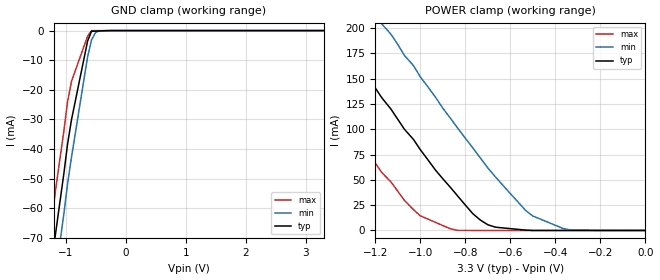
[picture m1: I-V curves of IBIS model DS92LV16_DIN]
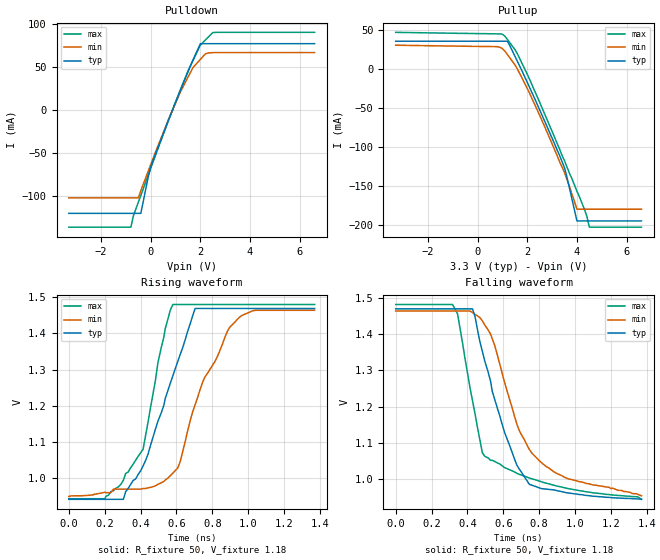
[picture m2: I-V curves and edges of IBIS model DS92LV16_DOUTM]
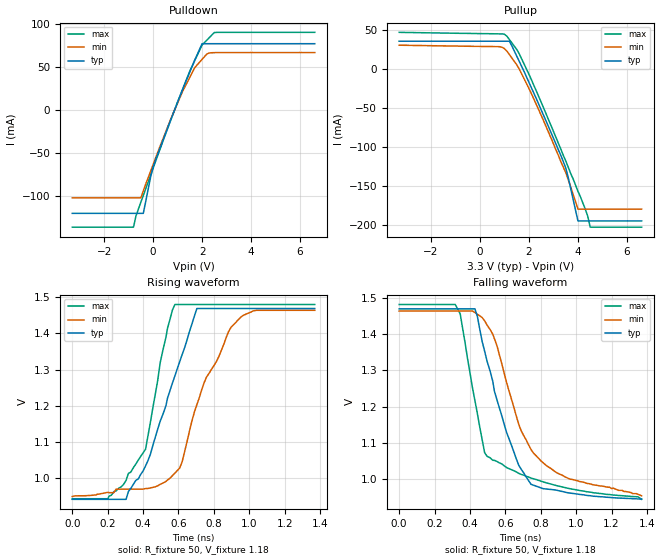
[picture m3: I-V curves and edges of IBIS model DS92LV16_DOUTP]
|   National Semiconductor Corporation
|   IBIS Model of DS92LV16TVHG
|   16-Bit BUS LVDS Serializer/Deserializer
|   80 Lead PQFP Package
[IBIS Ver]   3.2
[Comment Char]   |_char
[File name]   ds92lv16tvhg.ibs
[File Rev]   1.5
[Date]   03/22/04
[Source]
SPICE to IBIS Translation
[Notes]
Created by Tim Coyle; dglisic for Revs 1.4 and beyond.
Rev 1.5: - Updated RINP and RINM models.
Rev 1.4: - Changed Cref to 15pF, to match the datasheet value.
Rev 1.3: - Fixed V-T time scale for LVDS output data
   - Modified pull-up data for LVDS output data to make more accurate
   - Accounted for power/ground clamp data in output models
Rev 1.2: - Changed Ramp values in accordance with IBIS specification
Rev 1.1: - Changed RCLK and LOCK pins to output model types
   - Added typ min max description to Ramp data for clarification
[Disclaimer]
(C) Copyright National Semiconductor Corporation 2002
   All rights reserved
   National Semiconductor Corporation hereby grants
the user of this IBIS model a non-exclusive, nontransferable
license to use this IBIS model under the following terms.
Before using this IBIS model, the user should read this
license.  If the user does not accept these terms,  the
IBIS model should be returned to National within 30 days.
   The user is granted this license only to use the
IBIS model and is not granted rights to sell, load, rent,
lease or license the IBIS model in whole or in part, or in
modified form to anyone other than user. User may modify
the IBIS model to suit its specific applications but rights
to derivative works and such modifications shall belong to
National.
   This IBIS model is provided on an "AS IS" basis and
National makes absolutely no warranty with respect to the
information contained herein.NATIONAL DISCLAIMS AND CUSTOMER
WAIVES ALL WARRANTIES, EXPRESS OR IMPLIED, INCLUDING
WARRANTIES OF MERCHANTABILITY OR FITNESS FOR A PARTICULAR
PURPOSE. The entire risk as to quality and performance is
with the Customer. ACCORDINGLY, IN NO EVENT SHALL THE
COMPANY BE LIABLE FOR ANY DAMAGES, WHETHER IN CONTRACT OR
TORT,INCLUDING ANY LOST PROFITS OR OTHER INCIDENTAL,
CONSEQUENTIAL, EXEMPLARY, OR PUNITIVE DAMAGES ARISING OUT
OF THE USE OR APPLICATION OF THE IBIS model provided in
this package.Further, National reserves the right to make
changes without notice to any product herein to improve
reliability, function, or design. National does not convey
any license under patent rights or any other intellectual
property rights, including those of third parties.
   National is not obligated to provide maintenance or support
for the licensed IBIS model.
Contact National at ATTN:INTERFACE APPLICATIONS/IBIS MODELS.
5 Foden Road, M/S 03-03, South Porltand, ME 04106
(207) 541-8203
[Copyright]
(c) Copyright 2002 National Semiconductor Corp.
[Component]   DS92LV16
Si_location Pin
Timing_location Pin
[Manufacturer]   National Semiconductor Corp.
[Package]
|   TYP   MIN   MAX
R_pkg   50.0m   50.0m   50.0m
L_pkg   1.164nH   1.04n   1.33n
C_pkg   0.207pF   0.178p   0.245p
[Pin]   signal_name   model_name   R_pin   L_pin   C_pin
1   RPWDN   DS92LV16_CONTROL   50.0m   1.33n   0.245p
2   REN   DS92LV16_CONTROL   50.0m   1.04n   0.178p
3   CONFIG1 DS92LV16_CONTROL   50.0m   1.04n   0.178p
4   REFCLK  DS92LV16_CONTROL   50.0m   1.04n   0.178p
5   AVDD   POWER   50.0m   1.33n   0.245p
6   AGND   GND   50.0m   1.04n   0.178p
7   RINP   DS92LV16_RINP   50.0m   1.04n   0.178p
8   RINM   DS92LV16_RINM   50.0m   1.33n   0.245p
9   AGND   GND   50.0m   1.33n   0.245p
10   AVDD   POWER   50.0m   1.33n   0.245p
11   AVDD   POWER   50.0m   1.33n   0.245p
12   AGND   GND   50.0m   1.33n   0.245p
13   DOUTP   DS92LV16_DOUTP   50.0m   1.33n   0.245p
14   DOUTM   DS92LV16_DOUTM   50.0m   1.33n   0.245p
15   AVDD   POWER   50.0m   1.33n   0.245p
16   AGND   GND   50.0m   1.33n   0.245p
17   TCLK   DS92LV16_CONTROL   50.0m   1.33n   0.245p
18   CONFIG2 DS92LV16_CONTROL   50.0m   1.33n   0.245p
19   DEN   DS92LV16_CONTROL   50.0m   1.33n   0.245p
20   SYNC   DS92LV16_CONTROL   50.0m   1.33n   0.245p
21   DIN0   DS92LV16_DIN   50.0m   1.33n   0.245p
22   DIN1   DS92LV16_DIN   50.0m   1.33n   0.245p
23   DIN2   DS92LV16_DIN   50.0m   1.33n   0.245p
24   DIN3   DS92LV16_DIN   50.0m   1.33n   0.245p
25   DIN4   DS92LV16_DIN   50.0m   1.33n   0.245p
26   DIN5   DS92LV16_DIN   50.0m   1.33n   0.245p
27   DIN6   DS92LV16_DIN   50.0m   1.33n   0.245p
28   DIN7   DS92LV16_DIN   50.0m   1.33n   0.245p
29   PGND   GND   50.0m   1.33n   0.245p
30   PVDD   POWER   50.0m   1.33n   0.245p
31   PVDD   POWER   50.0m   1.33n   0.245p
32   PGND   GND   50.0m   1.33n   0.245p
33   DIN8   DS92LV16_DIN   50.0m   1.33n   0.245p
34   DIN9   DS92LV16_DIN   50.0m   1.33n   0.245p
35   DIN10   DS92LV16_DIN   50.0m   1.33n   0.245p
36   DIN11   DS92LV16_DIN   50.0m   1.33n   0.245p
37   DIN12   DS92LV16_DIN   50.0m   1.33n   0.245p
38   DIN13   DS92LV16_DIN   50.0m   1.33n   0.245p
39   DIN14   DS92LV16_DIN   50.0m   1.33n   0.245p
40   DIN15   DS92LV16_DIN   50.0m   1.33n   0.245p
41   DGND   GND   50.0m   1.33n   0.245p
42   TPWDN   DS92LV16_CONTROL   50.0m   1.33n   0.245p
43   DVDD   POWER   50.0m   1.33n   0.245p
44   DGND   GND   50.0m   1.33n   0.245p
45   ROUT0   DS92LV16_ROUT   50.0m   1.33n   0.245p
46   ROUT1   DS92LV16_ROUT   50.0m   1.33n   0.245p
47   ROUT2   DS92LV16_ROUT   50.0m   1.33n   0.245p
48   ROUT3   DS92LV16_ROUT   50.0m   1.33n   0.245p
49   RCLK   DS92LV16_ROUT   50.0m   1.33n   0.245p
50   DVDD   POWER   50.0m   1.33n   0.245p
51   DGND   GND   50.0m   1.33n   0.245p
52   DGND   GND   50.0m   1.33n   0.245p
53   DVDD   POWER   50.0m   1.33n   0.245p
54   ROUT4   DS92LV16_ROUT   50.0m   1.33n   0.245p
55   ROUT5   DS92LV16_ROUT   50.0m   1.33n   0.245p
56   ROUT6   DS92LV16_ROUT   50.0m   1.33n   0.245p
57   ROUT7   DS92LV16_ROUT   50.0m   1.33n   0.245p
58   DVDD   POWER   50.0m   1.33n   0.245p
59   DGND   GND   50.0m   1.33n   0.245p
60   DGND   GND   50.0m   1.33n   0.245p
61   DGND   GND   50.0m   1.33n   0.245p
62   DVDD   POWER   50.0m   1.33n   0.245p
63   LOCK   DS92LV16_ROUT   50.0m   1.33n   0.245p
64   ROUT8   DS92LV16_ROUT   50.0m   1.33n   0.245p
65   ROUT9   DS92LV16_ROUT   50.0m   1.33n   0.245p
66   ROUT10  DS92LV16_ROUT   50.0m   1.33n   0.245p
67   ROUT11  DS92LV16_ROUT   50.0m   1.33n   0.245p
68   DGND   GND   50.0m   1.33n   0.245p
69   DVDD   POWER   50.0m   1.33n   0.245p
70   ROUT12  DS92LV16_ROUT   50.0m   1.33n   0.245p
71   ROUT13  DS92LV16_ROUT   50.0m   1.33n   0.245p
72   ROUT14  DS92LV16_ROUT   50.0m   1.33n   0.245p
73   ROUT15  DS92LV16_ROUT   50.0m   1.33n   0.245p
74   PGND   GND   50.0m   1.33n   0.245p
75   PVDD   POWER   50.0m   1.33n   0.245p
76   PGND   GND   50.0m   1.33n   0.245p
77   PVDD   POWER   50.0m   1.33n   0.245p
78   LINELE  DS92LV16_CONTROL   50.0m   1.33n   0.245p
79   LOCALLE DS92LV16_CONTROL   50.0m   1.33n   0.245p
80   DGND   GND   50.0m   1.33n   0.245p
[Diff Pin] inv_pin   vdiff   tdelay_typ   tdelay_min   tdelay_max
| The '+' pin is Diff_pin and the '-' pin is the inv_pin
| Receiver Vth = +/-100mV
7   8   0.1   0   0   0
13   14   NA   0   0   0
| Models and submodels in the file (7): DS92LV16_DIN (Input), DS92LV16_DOUTM (Output), DS92LV16_DOUTP (Output), DS92LV16_RINM (Input), DS92LV16_RINP (Input), DS92LV16_ROUT (Output), DS92LV16_CONTROL (Input)
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[Model]   DS92LV16_DIN
Model_type Input
Vinh=2.0
Vinl=0.8
C_comp   2.922pF   2.922pF   2.922pF
[Temperature Range] 25   85   -40
[Voltage Range]   3.3   3.15   3.45
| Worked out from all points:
|   GND clamp passes 1 mA (typ) near -0.58 V on its own axis
|   POWER clamp passes 1 mA (typ) near -0.56 V on its own axis
[GND Clamp]
|V(groundclamp)   I(typ)   I(min)   I(max)
-3.3V     -416mA     -429mA     -402mA
-1.3V     -89.7mA    -104mA     -74.9mA
-1.23V    -79.3mA    -93mA      -64.5mA
-1.17V    -69.1mA    -82.7mA    -54.4mA
-1.1V     -58.8mA    -72.5mA    -44.3mA
-1.03V    -48.6mA    -62.2mA    -34.2mA
-967mV    -38.4mA    -51.9mA    -24.1mA
-900mV    -30mA      -42.6mA    -17.1mA
-633mV    -3.57mA    -8.92mA    -1.9mA
-567mV    -239uA     -3.14mA    -420nA
-433mV    -133uA     -61.9uA    -233nA
3.3V      21.4pA     6.6nA      19.4pA
[POWER Clamp]
|Vtable   I(typ)   I(min)   I(max)
-3.3V     826mA      900mA      750mA
-1.63V    280mA      354mA      203mA
-1.6V     269mA      344mA      193mA
-1.37V    194mA      268mA      118mA
-1.17V    131mA      204mA      57.1mA
-1.13V    120mA      194mA      48mA
-1V       80mA       152mA      14.5mA
-833mV    33.9mA     101mA      60uA
-700mV    5.68mA     61.9mA     6.68uA
-533mV    372uA      20mA       1.71nA
-366mV    1.1uA      2.03mA     12.8pA
0V        6.66pA     6.59nA     6.3pA
[Model]   DS92LV16_DOUTM
Model_type Output
Polarity Inverting
Vref=1.20
Vmeas=1.20
Rref=50   | 100 Ohms Across Outputs OUTP and OUTM
Cref=5p
C_comp   3.122pF   3.122pF   3.122pF
[Temperature Range] 25   85   -40
[Voltage Range]   3.3   3.15   3.45
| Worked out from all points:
|   slope of the pulldown table from 0 to 0.495 V, typ, clamps not added: 13.1 ohm
|   falling waveform, R_fixture 50, V_fixture 1.18: 20-80 % time 190ps typ, 235ps min, 166ps max; typ from 1.47 V to 0.945 V
|   rising waveform, R_fixture 50, V_fixture 1.18: 20-80 % time 210ps typ, 224ps min, 147ps max; typ from 0.942 V to 1.47 V
[Pullup]
|Vtable   I(typ)   I(min)   I(max)
-3.3V     35mA       29.9mA     46.4mA
800mV     35mA       28mA       44.4mA
1.1V      35mA       22.3mA     41.4mA
1.2V      35mA       18mA       37.2mA
1.6V      9.43mA     -402uA     19.1mA
2.4V      -45.7mA    -52.9mA    -36mA
3.3V      -111mA     -119mA     -103mA
3.5V      -127mA     -133mA     -118mA
4V        -195mA     -180mA     -157mA
4.4V      -195mA     -180mA     -189mA
4.5V      -195mA     -180mA     -203mA
6.6V      -195mA     -180mA     -203mA
[Pulldown]
|V(pulldown)   I(typ)   I(min)   I(max)
-3.3V     -120mA     -102mA     -136mA
-800mV    -120mA     -102mA     -136mA
-700mV    -120mA     -102mA     -123mA
-500mV    -120mA     -102mA     -107mA
-400mV    -120mA     -93.8mA    -99.3mA
0V        -66.3mA    -63.4mA    -67.5mA
1.2V      23.4mA     21.4mA     23.8mA
1.7V      58mA       49.2mA     57.4mA
2V        77mA       58.8mA     75.5mA
2.2V      77mA       65.2mA     81.3mA
2.5V      77mA       66.6mA     90mA
6.6V      77mA       66.7mA     90.2mA
[Ramp]
|   typ   min   max
dV/dt_r   320mV/.213ns   310mV/.222ns   330mV/.150ns
dV/dt_f   320mv/.192ns   310mv/.241ns   330mv/.156ns
R_load=50
[Falling Waveform]
R_fixture=50
V_fixture=1.18
V_fixture_min=1.18
V_fixture_max=1.18
0s        1.47V      1.464V     1.482V
317ps     1.47V      1.464V     1.482V
345ps     1.47V      1.464V     1.456V
428ps     1.47V      1.46V      1.217V
497ps     1.325V     1.425V     1.063V
607ps     1.129V     1.267V     1.032V
676ps     1.038V     1.151V     1.016V
745ps     985.7mV    1.082V     1.003V
966ps     961.6mV    1V         973.5mV
1.37ns    945mV      954mV      944.3mV
[Rising Waveform]
R_fixture=50
V_fixture=1.18
V_fixture_min=1.18
V_fixture_max=1.18
0s        941.6mV    949.5mV    943.3mV
202ps     941.6mV    961.1mV    943.3mV
304ps     941.6mV    969.8mV    994mV
414ps     1.034V     971.4mV    1.08V
497ps     1.158V     983.1mV    1.32V
580ps     1.283V     1.014V     1.48V
704ps     1.469V     1.203V     1.48V
897ps     1.469V     1.417V     1.48V
1.04ns    1.469V     1.464V     1.48V
1.37ns    1.469V     1.464V     1.48V
[Model]   DS92LV16_DOUTP
Model_type Output
Polarity Non-Inverting
Vref=1.20
Vmeas=1.20
Rref=50   | 100 Ohms Across Outputs OUTP and OUTM
Cref=5p
C_comp   3.122pF   3.122pF   3.122pF
[Temperature Range] 25   85   -40
[Voltage Range]   3.3   3.15   3.45
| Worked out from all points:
|   slope of the pulldown table from 0 to 0.495 V, typ, clamps not added: 13.1 ohm
|   falling waveform, R_fixture 50, V_fixture 1.18: 20-80 % time 190ps typ, 235ps min, 166ps max; typ from 1.47 V to 0.945 V
|   rising waveform, R_fixture 50, V_fixture 1.18: 20-80 % time 210ps typ, 224ps min, 147ps max; typ from 0.942 V to 1.47 V
[Pullup]
|Vtable   I(typ)   I(min)   I(max)
-3.3V     35mA       29.9mA     46.4mA
800mV     35mA       28mA       44.4mA
1.1V      35mA       22.3mA     41.4mA
1.2V      35mA       18mA       37.2mA
1.6V      9.43mA     -402uA     19.1mA
2.4V      -45.7mA    -52.9mA    -36mA
3.3V      -111mA     -119mA     -103mA
3.5V      -127mA     -133mA     -118mA
4V        -195mA     -180mA     -157mA
4.4V      -195mA     -180mA     -189mA
4.5V      -195mA     -180mA     -203mA
6.6V      -195mA     -180mA     -203mA
[Pulldown]
|V(pulldown)   I(typ)   I(min)   I(max)
-3.3V     -120mA     -102mA     -136mA
-800mV    -120mA     -102mA     -136mA
-700mV    -120mA     -102mA     -123mA
-500mV    -120mA     -102mA     -107mA
-400mV    -120mA     -93.8mA    -99.3mA
0V        -66.3mA    -63.4mA    -67.5mA
1.2V      23.4mA     21.4mA     23.8mA
1.7V      58mA       49.2mA     57.4mA
2V        77mA       58.8mA     75.5mA
2.2V      77mA       65.2mA     81.3mA
2.5V      77mA       66.6mA     90mA
6.6V      77mA       66.7mA     90.2mA
[Ramp]
|   typ   min   max
dV/dt_r   320mV/.213ns   310mV/.222ns   330mV/.150ns
dV/dt_f   320mv/.192ns   310mv/.241ns   330mv/.156ns
R_load=50
[Falling Waveform]
R_fixture=50
V_fixture=1.18
V_fixture_min=1.18
V_fixture_max=1.18
0s        1.47V      1.464V     1.482V
317ps     1.47V      1.464V     1.482V
345ps     1.47V      1.464V     1.456V
428ps     1.47V      1.46V      1.217V
497ps     1.325V     1.425V     1.063V
607ps     1.129V     1.267V     1.032V
676ps     1.038V     1.151V     1.016V
745ps     985.7mV    1.082V     1.003V
966ps     961.6mV    1V         973.5mV
1.37ns    945mV      954mV      944.3mV
[Rising Waveform]
R_fixture=50
V_fixture=1.18
V_fixture_min=1.18
V_fixture_max=1.18
0s        941.6mV    949.5mV    943.3mV
202ps     941.6mV    961.1mV    943.3mV
304ps     941.6mV    969.8mV    994mV
414ps     1.034V     971.4mV    1.08V
497ps     1.158V     983.1mV    1.32V
580ps     1.283V     1.014V     1.48V
704ps     1.469V     1.203V     1.48V
897ps     1.469V     1.417V     1.48V
1.04ns    1.469V     1.464V     1.48V
1.37ns    1.469V     1.464V     1.48V
